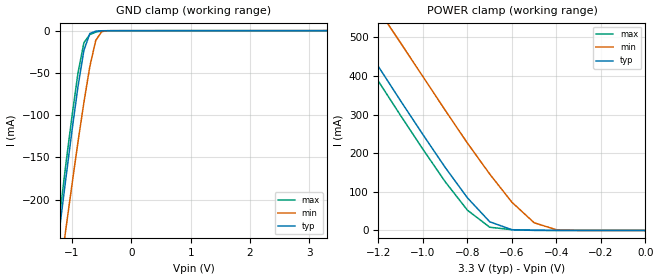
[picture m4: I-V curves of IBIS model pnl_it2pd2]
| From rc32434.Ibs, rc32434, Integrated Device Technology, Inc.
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[Model]   pnl_it2pd2
Model_type   Input
Polarity   Non-Inverting
Enable   Active-High
Vinl =  0.800V
Vinh =  2.000V
C_comp   0.40pF   0.30pF   0.50pF
[Temperature Range]   25.00   0.12k   0.000
[Voltage Range]   3.30V   3.00V   3.60V
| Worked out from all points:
|   GND clamp passes 1 mA (typ) near -0.62 V on its own axis
|   POWER clamp passes 1 mA (typ) near -0.55 V on its own axis
[GND_clamp]
| voltage   I(typ)   I(min)   I(max)
-3.3V     -1.469A    -1.42A     -1.487A
-1.3V     -286mA     -337mA     -272mA
-1.2V     -229mA     -285mA     -214mA
-1.1V     -173mA     -233mA     -156mA
-1V       -118mA     -182mA     -101mA
-900mV    -66.54mA   -132mA     -50.37mA
-800mV    -23.33mA   -85.13mA   -14.25mA
-700mV    -3.36mA    -42.49mA   -4.639mA
-600mV    -569uA     -11.57mA   -1.694mA
-500mV    -87.97uA   -1.105mA   -340uA
-300mV    -13.58uA   -11.55uA   -18.14uA
3.3V      49.8uA     126uA      75.12uA
[POWER_clamp]
| voltage   I(typ)   I(min)   I(max)
-3.3V     2.292A     2.4A       2.265A
-1.4V     601mA      745mA      565mA
-1.3V     513mA      658mA      475mA
-1.2V     424mA      571mA      386mA
-1.1V     335mA      485mA      297mA
-900mV    163mA      311mA      126mA
-800mV    84.3mA     226mA      52.37mA
-700mV    22.58mA    146mA      8.427mA
-600mV    1.806mA    72.93mA    1.995mA
-500mV    238uA      19.89mA    664uA
-400mV    67uA       1.844mA    156uA
0V        0A         0A         0A
